PROGRAM MAIN
VAR
	Axis_Master			: Axis_ref;			//定义主轴
	Axis_Slave			: Axis_ref;			//定义从轴
	Master_Power		: MC_Power;			//主轴使能
	Slave_Power			: MC_Power;			//从轴使能
	Master_Calibrate	: MC_Jog;			//主轴点动
	Slave_Calibrate		: MC_Jog;			//从轴点动
	Axes_GearIn			: MC_GearInDyn;		//动态耦合
	Master_Move			: MC_MoveVelocity;	//主轴运动
	Axes_GearOut		: MC_GearOut;		//从轴解耦
	Master_Stop			: MC_Stop;			//主轴停止
	Slave_Stop			: MC_Stop;			//从轴停止

	iState				: INT:= 0;			//程序状态机
	rRatio				: LREAL:=-1;		//耦合系数
	bSwitch_1			: BOOL;				//切换耦合系数按钮1
	bSwitch_2			: BOOL;				//切换耦合系数按钮2
	bSwitch_3			: BOOL;				//切换耦合系数按钮3
	bGearIn				: BOOL;				//耦合按钮
	bStart				: BOOL;				//启动按钮
	bGearOut			: BOOL;				//解耦按钮	
	bStop				: BOOL;				//停止按钮
	
	EL1008_1	AT%I*	: BOOL;				//按钮1，正转点动
	EL1008_2	AT%I*	: BOOL;				//按钮2，反转点动
	EL1008_3	AT%I*	: BOOL;				//按钮3，切换需要点动的轴
	EL3255_1	AT%I*	: INT;				//电位器，调节主轴转速
	
END_VAR

CASE iState	OF
	Powering_Axes:							//运行程序自动使能两轴
		Master_Power.Enable			:= TRUE;
		Slave_Power.Enable			:= TRUE;
		IF Master_Power.Active AND Slave_Power.Active THEN
			iState					:= Calibrating_Master;
		END_IF
		
	Calibrating_Master:						//点动主轴,调整位置
		Master_Calibrate(
			Axis					:= Axis_Master, 
			JogForward				:= EL1008_1, 
			JogBackwards			:= EL1008_2, 
			Mode					:= 2, 
			Velocity				:= 15, 
			);
		IF EL1008_3 THEN
			iState					:= Calibrating_Slave;
		END_IF
		
	Calibrating_Slave:						//点动从轴,调整位置
		Slave_Calibrate(
			Axis					:= axis_slave,
			JogForward				:= EL1008_1,
			JogBackwards			:= EL1008_2,
			Mode					:= 2, 
			Velocity				:= 15,
			);	
		IF bGearIn THEN
			istate					:= Gearin_Axes;
		END_IF

	Gearin_Axes:							//电机转动前,执行耦合
		Axes_GearIn.Enable			:= TRUE;
		IF Axes_GearIn.InGear AND bStart THEN
			iState					:= Moving_Master;
		END_IF
		
	Moving_Master:							//主轴转动
		Master_Move.Execute			:= TRUE;
		IF Master_Move.InVelocity THEN
			Master_Move.Execute		:= FALSE;
		END_IF
		IF bGearOut THEN
			Axes_GearIn.Enable		:= FALSE;
			Master_Move.Execute		:= FALSE;
			iState					:= GearOut_Axes;
		END_IF
		
	GearOut_Axes:							//执行解耦
		Axes_GearOut.Execute		:= TRUE;
		IF Axes_GearOut.Done THEN
			Axes_GearOut.Execute	:= FALSE;	
		END_IF
		IF bStop THEN
			iState					:= Stopping_Axes;
		END_IF
		
	Stopping_Axes:							//停止转动
		Master_Stop.Execute			:= TRUE;
		Slave_Stop.Execute			:= TRUE;
		IF Master_Stop.Done AND Slave_Stop.Done THEN
			Master_Stop.Execute		:= FALSE;
			Slave_Stop.Execute		:= FALSE;
			Master_Move.Execute		:= FALSE;
			iState					:= Calibrating_Master;
		END_IF

END_CASE
Power_Axes();								//调用使能功能块
Gear_Axes();								//调用耦合解耦功能块
Move_Axes();								//调用轴运动功能块
Stop_Axes();								//调用停止功能块
Switch_Ratio();								//切换耦合系数

ACTION Gear_Axes:
Axes_GearIn(
	Master := Axis_Master,
	Slave := axis_Slave,
	GearRatio := rRatio,
	Acceleration:= 15000, 
	Deceleration:= 15000,	
	Ingear	=> 
	);
Axes_GearOut(
	Slave:= Axis_Slave, 
	Done=>  
	 );
END_ACTION

ACTION Move_Axes:
Master_Move(
	Axis	:= Axis_Master,
	Velocity:= EL3255_1/100,
	Direction	:= 3,
	InVelocity	=> 
	);
END_ACTION

ACTION Power_Axes:
Master_Power(
	Axis:= Axis_Master,  
	Enable_Positive:= TRUE, 
	Enable_Negative:= TRUE, 
	Override:= 100, 
	Active=> , 
	 );
Slave_Power(
	Axis:= Axis_Slave,  
	Enable_Positive:= TRUE, 
	Enable_Negative:= TRUE, 
	Override:= 100, 
	Active=> , 
	 );
END_ACTION

ACTION Stop_Axes:
Master_Stop(
	Axis:= Axis_Master, 
	Done=> 
	 );
Slave_Stop(
	Axis:= Axis_Slave, 
	Done=> 
	 );
END_ACTION

ACTION Switch_Ratio:
IF	bSwitch_1 THEN
	rRatio		:= -1;
ELSIF bSwitch_2 THEN
	rRatio		:= -2;
ELSIF bSwitch_3 THEN
	rRatio		:= -10;
END_IF
END_ACTION

END_PROGRAM
